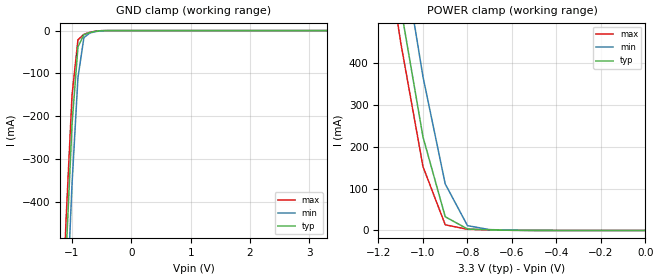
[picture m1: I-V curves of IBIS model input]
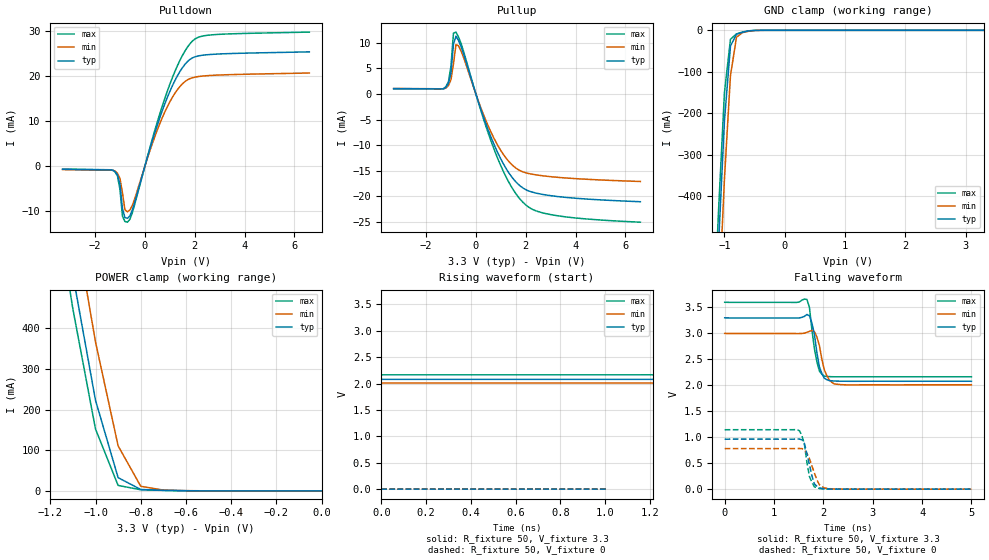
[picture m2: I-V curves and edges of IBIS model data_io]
| SOJ package &   Commercial  Operation
[IBIS Ver]   3.2
[Comment Char]   |_char
[File name]   as7c31024b_sojc.ibs
[File Rev]   1.0
[Date]   Jun 9, 2004 2:17:37 PM
[Source]
Alliance Semiconductor Corporation
[Notes]
This model  is for SOJ package &
 Commercial  Operation
[Disclaimer]
Data is for modeling purpose only and is not guaranted.
This IBIS model is provided on an "AS IS" basis and Alliance Semiconductor makes
absolutely no warranty with respect to the information contained
herein.The entire risk as to quality and performance
is with the Customer. ACCORDINGLY, IN NO EVENT SHALL THE COMPANY BE
LIABLE FOR ANY DAMAGES, WHETHER IN CONTRACT OR TORT,INCLUDING ANY
LOST PROFITS OR OTHER INCIDENTAL, CONSEQUENTIAL, EXEMPLARY, OR
PUNITIVE DAMAGES ARISING OUT OF THE USE OR APPLICATION OF THE IBIS
model provided in this package.
[Copyright]
Alliance Semiconductor Corporation
| SOJ Package & Commercial Operation.
[Component]   AS7C31024B_SOJC
Si_location Pin
Timing_location Pin
[Manufacturer]   Alliance Semiconductor Corporation
[Package]
R_pkg   351.65m   239.7m   463.6m
L_pkg   8.523nH   5.387nH   11.66nH
C_pkg   1.885pF   1.215pF   2.556pF
[Pin] signal_name   model_name
1   NC   NC
2   A16   input
3   A14   input
4   A12   input
5   A7   input
6   A6   input
7   A5   input
8   A4   input
9   A3   input
10   A2   input
11   A1   input
12   A0   input
13   IO0   data_io
14   IO1   data_io
15   IO2   data_io
16   GND   GND
17   IO3   data_io
18   IO4   data_io
19   IO5   data_io
20   IO6   data_io
21   IO7   data_io
22   NCE1   input
23   A10   input
24   NOE   input
25   A11   input
26   A9   input
27   A8   input
28   A13   input
29   NWE   input
30   NCE2   input
31   A15   input
32   VCC   POWER
| Models and submodels in the file (2): input (Input), data_io (I/O)
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[Model]   input
Model_type Input
Vinh=2V
Vinl=0.8V
C_comp   4pF   4pF   4pF
[Model Spec]
[Temperature Range] 25   70   0
[Voltage Range]   3.3   3.0   3.6
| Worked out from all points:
|   GND clamp passes 1 mA (typ) near -0.56 V on its own axis
|   POWER clamp passes 1 mA (typ) near -0.65 V on its own axis
[GND Clamp]
-3.3V     -8.605A    -8.678A    -8.569A
-1.2V     -871.8mA   -1.032A    -786.6mA
-1.1V     -525.3mA   -681.9mA   -442.6mA
-1V       -219.6mA   -359.8mA   -151.4mA
-900mV    -38.16mA   -110mA     -21.74mA
-800mV    -9.652mA   -16.68mA   -8.786mA
-700mV    -4.621mA   -5.631mA   -4.129mA
-600mV    -1.581mA   -2.258mA   -1.211mA
-400mV    -22.59uA   -71.08uA   -10.05uA
3.3V      156pA      1.566uA    81.03pA
[POWER Clamp]
-3.3V     8.613A     8.687A     8.576A
-1.2V     879.9mA    1.042A     793.6mA
-1.1V     531.7mA    690.5mA    447.6mA
-1V       222.9mA    366.4mA    152.1mA
-900mV    32.63mA    110.9mA    13.56mA
-800mV    3.618mA    11.48mA    2.851mA
-700mV    1.463mA    2.037mA    1.288mA
0V        156pA      1.542nA    96.3pA
[Model]   data_io
Model_type I/O
Enable Active-High
Polarity Non-Inverting
Vinh=2V
Vinl=0.8V
Vref=1.728V
Vmeas=1.5V
Rref=168
Cref=30pF
C_comp   4pF   4pF   4pF
[Temperature Range] 25   70   0
[Voltage Range]   3.3   3.0   3.6
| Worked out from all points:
|   slope of the pulldown table from 0 to 0.495 V, typ, clamps not added: 54.6 ohm
|   slope of the pullup table from 0 to 0.495 V, typ, clamps not added: 70.3 ohm
|   GND clamp passes 1 mA (typ) near -0.56 V on its own axis
|   POWER clamp passes 1 mA (typ) near -0.65 V on its own axis
|   falling waveform, R_fixture 50, V_fixture 3.3: 20-80 % time 132ps typ, 153ps min, 130ps max; typ from 3.3 V to 2.08 V
|   falling waveform, R_fixture 50, V_fixture 0: 20-80 % time 145ps typ, 183ps min, 125ps max; typ from 0.964 V to 0.002 V
|   rising waveform, R_fixture 50, V_fixture 3.3: 20-80 % time 130ps typ, 130ps min, 144ps max; typ from 2.08 V to 3.3 V
[Pullup]
-3.3V     1.05mA     1.087mA    1.024mA
-1.2V     1.343mA    1.17mA     1.474mA
-1.1V     2.093mA    1.672mA    2.412mA
-1V       4.162mA    2.808mA    5.487mA
-900mV    9.749mA    5.896mA    11.9mA
-800mV    11.31mA    9.656mA    12.11mA
-600mV    9.355mA    8.459mA    9.96mA
800mV     -10.66mA   -9.352mA   -11.68mA
1.4V      -15.96mA   -13.6mA    -17.92mA
1.9V      -18.41mA   -15.25mA   -21.23mA
3.1V      -19.94mA   -16.21mA   -23.66mA
6.6V      -21.06mA   -17.1mA    -25.06mA
[Pulldown]
-3.3V     -660uA     -727uA     -611uA
-1.2V     -1.16mA    -1.035mA   -1.221mA
-1V       -3.903mA   -2.651mA   -5.08mA
-900mV    -9.341mA   -5.846mA   -11.03mA
-800mV    -11.4mA    -9.637mA   -12.26mA
-700mV    -11.53mA   -10.09mA   -12.4mA
-500mV    -9.671mA   -8.648mA   -10.25mA
300mV     5.674mA    5.038mA    6.069mA
900mV     15.26mA    13.21mA    16.66mA
1.4V      20.98mA    17.67mA    23.43mA
1.9V      24.04mA    19.64mA    27.76mA
6.6V      25.41mA    20.71mA    29.8mA
[GND Clamp]
-3.3V     -8.605A    -8.678A    -8.569A
-1.2V     -871.7mA   -1.032A    -786.5mA
-1.1V     -525.2mA   -681.8mA   -442.5mA
-1V       -219.5mA   -359.7mA   -151.2mA
-900mV    -37.94mA   -109.8mA   -21.51mA
-800mV    -9.536mA   -16.55mA   -8.686mA
-700mV    -4.587mA   -5.581mA   -4.103mA
-600mV    -1.576mA   -2.248mA   -1.208mA
-400mV    -22.59uA   -71.06uA   -10.05uA
3.3V      156pA      1.566uA    81.03pA
[POWER Clamp]
-3.3V     8.613A     8.687A     8.576A
-1.2V     879.9mA    1.042A     793.6mA
-1.1V     531.7mA    690.5mA    447.6mA
-1V       222.9mA    366.4mA    152.1mA
-900mV    32.6mA     110.9mA    13.53mA
-800mV    3.604mA    11.47mA    2.839mA
-700mV    1.459mA    2.032mA    1.285mA
0V        156pA      1.542nA    96.3pA
[Falling Waveform]
R_fixture=50
V_fixture=3.3
V_fixture_min=3.0
V_fixture_max=3.6
0s        3.3V       3V         3.6V
1.667ns   3.365V     3.022V     3.654V
1.717ns   3.34V      3.039V     3.502V
1.768ns   3.198V     3.059V     3.071V
1.869ns   2.627V     2.931V     2.454V
1.919ns   2.357V     2.766V     2.275V
2.02ns    2.136V     2.296V     2.176V
2.121ns   2.092V     2.104V     2.169V
2.273ns   2.082V     2.022V     2.166V
5ns       2.079V     2.01V      2.166V
[Falling Waveform]
R_fixture=50
V_fixture=0
V_fixture_min=0
V_fixture_max=0
0s        963.8mV    781.9mV    1.146V
1.515ns   965.2mV    784.2mV    1.125V
1.566ns   952.3mV    782.5mV    1.032V
1.616ns   879.7mV    758.3mV    859.2mV
1.667ns   680.3mV    686.1mV    515mV
1.717ns   474.8mV    590.5mV    247.7mV
1.818ns   102.7mV    312.3mV    47.11mV
1.919ns   26.61mV    86.24mV    13.35mV
2.222ns   2.571mV    4.8mV      2.253mV
5ns       2.006mV    1.927mV    2.127mV
[Rising Waveform]
R_fixture=50
V_fixture=3.3
V_fixture_min=3.0
V_fixture_max=3.6
0s        2.079V     2.01V      2.165V
1.364ns   2.07V      2.007V     2.153V
1.414ns   2.108V     2.013V     2.244V
1.515ns   2.478V     2.156V     2.929V
1.566ns   2.831V     2.47V      3.218V
1.616ns   3.09V      2.719V     3.431V
1.717ns   3.202V     2.906V     3.524V
1.818ns   3.256V     2.933V     3.579V
2.172ns   3.298V     2.997V     3.598V
5ns       3.298V     2.998V     3.598V
[Rising Waveform]
R_fixture=50
V_fixture=0
V_fixture_min=0
V_fixture_max=0
0s        0V         0V         0V
50.51ps   896.1uV    848.8uV    954.9uV
101ps     1.777mV    1.684mV    1.894mV
202ps     2.077mV    1.983mV    2.203mV
505.1ps   1.921mV    1.842mV    2.032mV
606.1ps   1.931mV    1.852mV    2.043mV
707.1ps   1.978mV    1.895mV    2.094mV
909.1ps   1.993mV    1.909mV    2.11mV
1.01ns    1.991mV    1.906mV    2.108mV
